PROGRAM MAIN
VAR
	//Sample 01 and 02
	nCounter     AT %MD0 :DWORD;
	TP_1		: TP;
	TOGGEL		: BOOL;

	//Sample03
	 boolVal   : BOOL;
	 intVal    : INT;
	 dintVal   : DINT;
	 sintVal   : SINT;
	 lrealVal  : LREAL;
	 realVal   : REAL;
	 stringVal : STRING(20);
	 
	 myComplexStruct : MyComplexStruct;
	 
	//Sample10
	text : STRING[30] := 'Hello TwinCAT';
	
	//Sample11
	Time1:TIME := T#21H33M23S231MS;
    Date1:DT:=DT#1993-06-12-15:36:55.40;
	
	//Sample12
	PLCArray : ARRAY [0..99] OF INT;
  	Index: BYTE;
	
	//Sample13
	PLCStruct : PLCStruct;	
	
	//Sample14
	(*primitive Types*)
	bool1:BOOL := FALSE;
	int1:INT := 30000;
	dint1:DINT:=125000;
	usint1:USINT:=200;
	real1:REAL:= 1.2;
	lreal1:LREAL:=3.5;

	(*string Types*)
	str1:STRING := 'this is a test string';
	str2:STRING(5) := 'hallo';

	(*struct Types*)
	complexStruct1 : TComplexStruct;
	
	//Sample22
	uintValue 	: UDINT 	:= 54321;
	boolValue	: BOOL 		:= TRUE;
	dintValue	: DINT		:= -12345678;
	
	//Sample30
//	fbMath	: FB_MATH;
	TON1: TON;
	
		FbUPS: FB_S_UPS_CX51x0;
		
	SPDM_2PASS: E_PersistentMode;
	
	fbwtpers:FB_WritePersistentData;

	wttrig: BOOL;
	rtirg11: R_TRIG;
//	flash1: FB_Flash;
	ntshutdown: NT_Shutdown;
	tcstop: TC_Stop;
END_VAR

VAR PERSISTENT
	
	cnt :INT;
	

END_VAR



//Sample 01 and 02
nCounter := nCounter + 1;

//Sample 03
sintVal := sintVal + 1;
dintVal := dintVal + 5;
realVal := realVal + 0.1;
lrealVal := lrealVal + 0.1;

boolVal := FALSE;
TON1(IN:= TRUE, PT:= T#200MS, Q=> boolVal);
IF boolVal THEN
	IF intval > 12 THEN
		intval := 0;
	END_IF
	intVal := intVal + 1;
	stringVal := LEFT(Text, intVal);
	TON1(IN:= FALSE);
END_IF

//Sample12
FOR Index := 0 TO 99 DO
  PLCArray[Index] := 3500 + INDEX;
END_FOR

myComplexStruct.a := TRUE;




//flash1(tiTime_On:=T#10MS , tiTime_Off:=T#10MS , bFlash=> );
rtirg11(CLK:=FbUPS.bPowerFailDetect , Q=> );
	IF rtirg11.Q THEN
		cnt :=cnt +1;
	END_IF






FbUPS(
 sNetID:='' , 
 iPLCPort:=851 , 
 iUPSPort:=16#588 , 
 tTimeout:=DEFAULT_ADS_TIMEOUT, 
 eUpsMode:=eSUPS_WrPersistData_NoShutdown ,//eSUPS_WrPersistData_Shutdown,  eSUPS_CheckPowerStatus   eSUPS_WrPersistData_NoShutdown  eSUPS_ImmediateShutdown
 ePersistentMode:=SPDM_2PASS   ,//SPDM_2PASS,   SPDM_VAR_BOOST
 tRecoverTime:=T#1S, 
 bPowerFailDetect=> , 
 eState=> );
 
 (*

	
	ntshutdown(
	NETID:='' , 
	DELAY:=0 , 
	START:=FbUPS.bPowerFailDetect  , 
	TMOUT:=T#5S , 
	BUSY=> , 
	ERR=> , 
	ERRID=> );
	
*)	

	
	tcstop(
	NETID:='' , 
	STOP:=FbUPS.bPowerFailDetect , 
	TMOUT:=T#1S , 
	BUSY=> , 
	ERR=> , 
	ERRID=> );
	











	
	

(*	
 fbwtpers(
	NETID:='' , 
	PORT:=851 , 
	START:= flash1.bFlash , 
	TMOUT:=T#2S , 
	MODE:= , 
	BUSY=> , 
	ERR=> , 
	ERRID=> );
*)

END_PROGRAM
